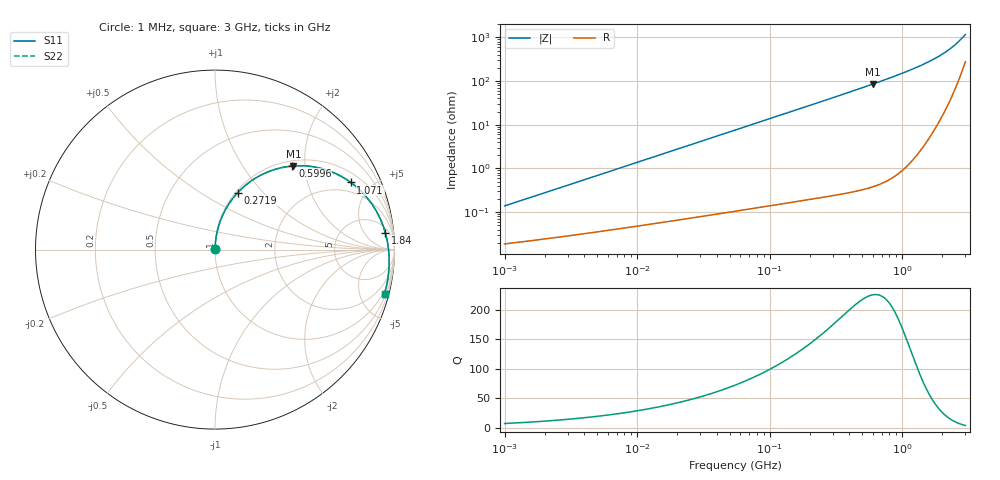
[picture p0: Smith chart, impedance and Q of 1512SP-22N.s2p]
# MHz  S  MA  R  50
!Freq  MagS11  AngS11  MagS21  AngS21  MagS12  AngS12  MagS22  AngS22
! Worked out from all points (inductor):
!   801 points, 1 MHz to 3 GHz, reference 50 ohm
!   read as one part in series: L = 21.9 nH near 1.041 MHz
!   highest Q = 225 at 605.6 MHz (marker M1), where L = 22.6 nH
!   S11 on the Smith chart (normalised r, x): 1 MHz: 1.00, +0.00; 271.9 MHz: 1.02, +0.73; 599.6 MHz: 1.11, +1.73; 1.071 GHz: 1.44, +3.76; 1.84 GHz: 8, +16; 3 GHz: 0.73, -7.71
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1  0.001343 81.9  0.9998 -0.1  0.9998 -0.1  0.001343 81.9
3.824029  0.005096 86.1  0.9997 -0.3  0.9997 -0.3  0.005096 86.1
14.47755  0.01926 87.1  0.9993 -1.2  0.9993 -1.2  0.01925 87.1
30.36588  0.04035 86.4  0.9984 -2.5  0.9984 -2.5  0.04034 86.4
54.81117  0.07269 84.7  0.9963 -4.5  0.9963 -4.5  0.07268 84.7
111.5625  0.1468 80.4  0.9877 -9.0  0.9877 -9.0  0.1468 80.4
209.5995  0.2692 72.9  0.9612 -16.7  0.9612 -16.7  0.2691 72.9
271.9047  0.3416 68.3  0.9377 -21.4  0.9377 -21.4  0.3415 68.3
332.1698  0.4069 63.9  0.9112 -25.7  0.9112 -25.7  0.4068 63.9
401.7505  0.476 59.2  0.8771 -30.5  0.8771 -30.5  0.4758 59.2
500.7192  0.5622 52.9  0.8244 -36.8  0.8244 -36.8  0.562 52.9
599.5748  0.635 47.2  0.7697 -42.6  0.7697 -42.6  0.6348 47.2
605.6065  0.6391 46.8  0.7663 -42.9  0.7663 -42.9  0.6388 46.8
793.5315  0.7444 37.4  0.6643 -52.3  0.6643 -52.3  0.744 37.4
922.0867  0.7973 31.9  0.5995 -57.7  0.5995 -57.7  0.7969 31.9
1071.468  0.8442 26.3  0.5306 -63.3  0.5306 -63.3  0.8438 26.3
1418.078  0.9129 15.7  0.3972 -73.6  0.3972 -73.6  0.9124 15.7
1839.614  0.9535 5.7  0.2755 -82.7  0.2755 -82.7  0.9531 5.7
2095.27  0.9659 0.6  0.2179 -86.8  0.2179 -86.8  0.9656 0.6
2362.686  0.9731 -4.3  0.1678 -89.9  0.1678 -89.9  0.9729 -4.3
2585.417  0.9759 -8.0  0.1329 -91.5  0.1329 -91.5  0.9759 -8.0
3000  0.9762 -14.6  0.08256 -90.7  0.08256 -90.7  0.9766 -14.7
